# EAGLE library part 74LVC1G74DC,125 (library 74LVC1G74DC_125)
74LVC1G74 - Single D-type flip-flop with set and reset; positive edge trigger@en-us Source: Datasheet
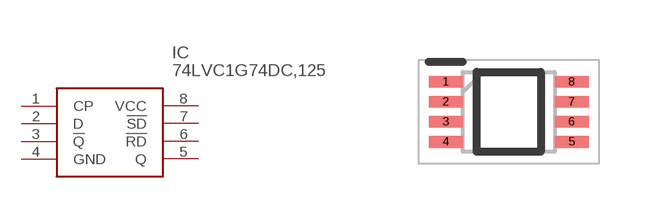
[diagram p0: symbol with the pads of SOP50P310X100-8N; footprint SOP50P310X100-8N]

Designator prefix IC

## 74LVC1G74DC,125 (Description: 74LVC1G74 - Single D-type flip-flop with set and reset; positive edge trigger@en-us; Height: 1mm; Manufacturer_Name: Nexperia; Manufacturer_Part_Number: 74LVC1G74DC,125; Mouser_Part_Number: 771-74LVC1G74DC-G; Mouser_Price-Stock: https://www.mouser.co.uk/ProductDetail/Nexperia/74LVC1G74DC125?qs=me8TqzrmIYWEN%2F9DZPyJbg%3D%3D)  [SOP50P310X100-8N]
1  CP
2  D
3  !Q
4  GND
5  Q
6  !RD
7  !SD
8  VCC

## Footprint SOP50P310X100-8N (pad centres in mm)
SOT765-1
smd 0.85 x 0.3: 1 -1.575,0.75; 2 -1.575,0.25; 3 -1.575,-0.25; 4 -1.575,-0.75; 5 1.575,-0.75; 6 1.575,-0.25; 7 1.575,0.25; 8 1.575,0.75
